{attribute 'no_assign'}
FUNCTION_BLOCK FB_IEDClient IMPLEMENTS I_ScsmAbortIndEventSink, I_ScsmAssociateCnfEventSink, I_ScsmGetServerDirectoryCnfEventSink, I_ScsmGetLogicalDeviceDirectoryCnfEventSink, I_ScsmGetLogicalNodeDirectoryCnfEventSink, I_ScsmGetDataValuesCnfEventSink, I_ScsmSetDataValuesCnfEventSink, I_ScsmReportIndEventSink, I_ScsmControlCnfEventSink, I_ScsmLastApplErrorIndEventSink, I_ScsmCommandTerminationIndEventSink
VAR_INPUT
	fbConnection		: FB_iec61850ClientClass := (ipAbortInd:=THIS^, ipAssociateCnf:=THIS^, ipGetServerDirectoryCnf:=THIS^, ipGetLogicalDeviceDirectoryCnf:=THIS^, ipGetLogicalNodeDirectoryCnf:=THIS^, ipGetDataValuesCnf:=THIS^, ipSetDataValuesCnf:=THIS^, ipReportInd:=THIS^, ipControlCnf:=THIS^, ipLastApplErrorInd:=THIS^, ipCommandTerminationInd:=THIS^);
END_VAR
VAR
	_bAbort				: BOOL; (* Rising edge activates AbortReq() command execution *)
	_bDisconnect		: BOOL; (* Rising edge activates ReleaseReq() command execution *)
	_bConnect			: BOOL; (* Rising edge activates AssociateReq() command execution *)
	_bReconnect			: BOOL := TRUE; (* TRUE => reconnect automatically *)
	_bReadAllData		: BOOL := TRUE; (* TRUE => read/refresh all data values on reconnect *)
	
	state				: BYTE;
	eState				: E_AsyncEnvironmentState; (* Environment state *)
	eLinkStatus			: E_ScsmLinkStatus; (* Network adapter link status *)
	bBusy				: BOOL; (* If TRUE => command execution is busy *)
	bSuccess			: BOOL;
	ipResult			: I_AsyncServiceResultClass;
	sLastErrorResult	: T_MaxString;
	fbAbortReason		: FB_ServiceErrorClass := (stError:=SUCCESS_EVENT);
	sLastAbortReason	: T_MaxString;
	nInvokeID			: UDINT;
	eServiceError		: E_AcsiServiceError; (* Latest OnXyzCnf() or OnXyzInd() event handler error *)
	nServiceError		: UDINT; (* Counts OnXyzCnf() and OnXyzInd() event handler errors *)
	nCmdError			: UDINT; (* Counts xyzReq() command errors *)
	sObjReference		: T_AcsiObjectReference; (* DATA object reference *)
	sCtrlReference		: T_AcsiObjectReference; (* CONTROLLABLE-DATA object reference *)
	
	bGetServerDirectory				: BOOL := TRUE; (* Rising edge enumerates logical-devices *)
	bGetLogicalDeviceDirectory		: BOOL := TRUE; (* Rising edge enumerates logical-nodes *)
	bGetLogicalNodeDirectory		: BOOL := TRUE; (* Rising edge enumerates "IEDMUnn/LLN0" data-sets *)
	bGetAllServerValues				: BOOL := TRUE; (* Rising edge reads all "IED" data attribute values *)
	bGetAllDataValues_LLN0_ST		: BOOL := TRUE; (* Rising edge reads all "IEDMUnn/LLN0.ST" data attribute values (having selected functional constraint) *)
	bGetDataValues_LLN0_ST_Beh		: BOOL := TRUE; (* Rising edge reads all "IEDMUnn/LLN0.ST.Beh" data attribute values (having selected functional constraint) *)
END_VAR

fbConnection.Execute();
eState:= fbConnection.eState;
eLinkStatus:= fbConnection.eLinkStatus;

CASE state OF
	0: (* Initial state *)
		IF _bAbort THEN (* Abort connection => execute AbortReq() command *)
			_bAbort:= FALSE;
			bSuccess:= fbConnection.AbortReq(ipReason:=fbAbortReason, ipSink:=0, ipResult=>ipResult);
			state:= SEL(bSuccess, 100, 1);
		ELSIF eState = E_AsyncEnvironmentState.Idle AND (_bConnect OR _bReconnect) THEN (* Open/establish connection => execute AssociateReq() command *)
			_bConnect:= FALSE;
			bGetAllServerValues:= SEL(_bReadAllData, bGetAllServerValues, TRUE);
			bSuccess:= fbConnection.AssociateReq(ipSink:=0, ipResult=>ipResult);
			state:= SEL(bSuccess, 100, 1);
		ELSIF eState = E_AsyncEnvironmentState.Established AND _bDisconnect THEN (* Close/release connection => execute ReleaseReq() command *)
			_bDisconnect:= FALSE;
			bSuccess:= fbConnection.ReleaseReq(ipSink:=0, ipResult=>ipResult);
			state:= SEL(bSuccess, 100, 1);
		ELSIF eState = E_AsyncEnvironmentState.Established THEN (* Connection established => exchange IED data *)
			state:= 10;
		END_IF
		_bConnect:= FALSE;
		_bDisconnect:= FALSE;
		(*==================================================================================================================================================================*)
	1: (* Wait for AbortReq() or ReleaseReq() or AssociateReq() command completion *)
		IF ipResult <> 0 THEN
			ipResult.Execute();
			IF NOT (bBusy:=ipResult.IsBusy()) THEN
				state:= SEL(ipResult.IsCompleted(), 100(* failed or aborted *), 0(* succeeded *));
			END_IF
		END_IF
		(*==================================================================================================================================================================*)
	10: (* Read/Write IED data *)
		IF bGetServerDirectory THEN (* Example => execute GetServerDirectoryReq() command *)
			bGetServerDirectory:= FALSE;
			bSuccess:= fbConnection.GetServerDirectoryReq(ipServer:=fbIED, eClass:=E_AcsiServerDirectoryClass.LogicalDevice, hUser:=0, ipSink:=0, nInvokeID=>nInvokeID, ipResult=>ipResult);
			state:= SEL(bSuccess, 100, 11);
		ELSIF bGetLogicalDeviceDirectory THEN (* Example => execute GetLogicalDeviceDirectoryReq() command *)
			bGetLogicalDeviceDirectory:= FALSE;
			bSuccess:= fbConnection.GetLogicalDeviceDirectoryReq(ipLogicalDevice:=fbIED.IEDMUnn, hUser:=0, ipSink:=0, nInvokeID=>nInvokeID, ipResult=>ipResult);
			state:= SEL(bSuccess, 100, 11);
		ELSIF bGetLogicalNodeDirectory THEN (* Example => execute GetLogicalNodeDirectoryReq() command *)
			bGetLogicalNodeDirectory:= FALSE;
			bSuccess:= fbConnection.GetLogicalNodeDirectoryReq(ipLogicalNode:=fbIED.IEDMUnn.LLN0, eClass:=E_AcsiLogicalNodeClass.DataSet, hUser:=0, ipSink:=0, nInvokeID=>nInvokeID, ipResult=>ipResult);
			state:= SEL(bSuccess, 100, 11);
		ELSIF bGetAllServerValues THEN (* Example => execute GetAllServerValues() command *)
			bGetAllServerValues:= FALSE;
			bSuccess:= fbConnection.GetAllServerValuesReq(ipServer:=fbIED, hUser:=0, ipSink:=0, nInvokeID=>nInvokeID, ipResult=>ipResult);
			state:= SEL(bSuccess, 100, 11);
		ELSIF bGetAllDataValues_LLN0_ST THEN (* Example => execute GetAllDataValuesReq() command *)
			bGetAllDataValues_LLN0_ST:= FALSE;
			bSuccess:= fbConnection.GetAllDataValuesReq(ipLogicalNode:=fbIED.IEDMUnn.LLN0, eFc:=E_AcsiFc.ST_, hUser:=0, ipSink:=0, nInvokeID=>nInvokeID, ipResult=>ipResult);
			state:= SEL(bSuccess, 100, 11);
		ELSIF bGetDataValues_LLN0_ST_Beh THEN (* Example => execute GetDataValuesReq() command *)
			bGetDataValues_LLN0_ST_Beh:= FALSE;
			bSuccess:= fbConnection.GetDataValuesReq(ipData:=fbIED.IEDMUnn.LLN0.Beh, eFc:=E_AcsiFc.ST_, hUser:=0, ipSink:=0, nInvokeID=>nInvokeID, ipResult=>ipResult);
			state:= SEL(bSuccess, 100, 11);
		ELSE
			state:= 0;
		END_IF
		(*==================================================================================================================================================================*)
	11: (* Wait for GetServerDirectoryReq(), GetLogicalDeviceDirectoryReq(), GetLogicalNodeDirectoryReq(), GetAllServerValuesReq(), GetAllDataValuesReq() or GetDataValuesReq() command completion *)
		IF ipResult <> 0 THEN
			ipResult.Execute();
			IF NOT (bBusy:=ipResult.IsBusy()) THEN
				state:= SEL(ipResult.IsCompleted(), 100(* failed or aborted *), 0(* succeeded *));
			END_IF
		END_IF
		(*==================================================================================================================================================================*)
	100: (* Error state *)
		state:= 0;
		IF ipResult <> 0 THEN
			nCmdError:= nCmdError + 1;
			sLastErrorResult:= ipResult.Dump();
		END_IF
END_CASE

PROPERTY bAbort : BOOL
SET
_bAbort:= bAbort;
END_SET
END_PROPERTY

PROPERTY bConnect : BOOL
SET
_bConnect:= bConnect;
END_SET
END_PROPERTY

PROPERTY bDisconnect : BOOL
SET
_bDisconnect:= bDisconnect;
END_SET
END_PROPERTY

PROPERTY bReconnect : BOOL
SET
_bReconnect:= bReconnect;
END_SET
END_PROPERTY

{attribute 'analysis' := '-33'}
(* This method receives IEC61850::Abort.ind primitive. *)
METHOD OnAbortInd
VAR_INPUT
	ipAA		: I_ScsmAssociationClass; (* Application association. If = 0 => optional. *)
	bPAbort		: BOOL; (* TRUE => P-Abort.request(), issued by provider, FALSE => Abort.request(), issued by user. *)
	ipReason	: I_ServiceErrorClass; (* Abort reason. *)
	ipData		: I_BaseStreamClass; (* Optional data. If = 0 => default, no data. *)
END_VAR
VAR
END_VAR
IF ipReason <> 0 THEN
	sLastAbortReason:= ipReason.Dump();
END_IF
END_METHOD

{attribute 'analysis' := '-33'}
(* This method receives IEC61850::Associate.cnf primitive. *)
METHOD OnAssociateCnf
VAR_INPUT
	ipAA			: I_ScsmAssociationClass; (* Application association. If = 0 => optional. *)
	eError			: E_AcsiServiceError; (* Error code *)
END_VAR
VAR
END_VAR
sLastAbortReason:= '';
sLastErrorResult:= '';
END_METHOD

{attribute 'analysis' := '-33'}
(* This method receives buffered IEC61850::Report.ind primitive. *)
METHOD OnBufferedReportInd
VAR_INPUT
	ipAA		: I_ScsmAssociationClass; (* Application association. If = 0 => optional. *)
	info		: ST_ScsmReportEventInfo;
	ipBrcb		: I_AcsiCommonBufferedReportControlBlockClass; (* Interface pointer to BRCB object. *)
	ipDataSet	: I_AcsiCommonDataSetClass; (* Interface pointer to data-set object. *)
	ipData		: I_AcsiCommonDataClass; (* Interface pointer to reported data object. *)
	eFc			: E_AcsiFc; (* Functional constraint of reported data. *)
	eError		: E_AcsiServiceError; (* Data access error code. *)
END_VAR
VAR
END_VAR
IF eError <> E_AcsiServiceError.NoError THEN
	eServiceError:= eError;
	nServiceError:= nServiceError + 1;
END_IF
IF ipData <> 0 THEN
	sObjReference:= ipData.GetObjectReference();
END_IF
END_METHOD

{attribute 'analysis' := '-33'}
(* This method receives IEC61850::CommandTermination.ind primitive. *)
METHOD OnCommandTerminationInd
VAR_INPUT
	ipAA		: I_ScsmAssociationClass; (* Application association. If = 0 => optional. *)
	info		: ST_ScsmCommandTerminationEventInfo;
	ipCtrl		: I_AcsiCommonControllableDataClass; (* Interface pointer to controllable data object. *)
	ipData		: I_AcsiCommonDataClass; (* Interface pointer to Oper/Cancel/SBO or SBOw data object. *)
	eFc			: E_AcsiFc; (* Functional constraint (CO). *)
	eError		: E_AcsiServiceError; (* Error code. *)
END_VAR
VAR
END_VAR
IF eError <> E_AcsiServiceError.NoError THEN
	eServiceError:= eError;
	nServiceError:= nServiceError + 1;
END_IF
IF ipCtrl <> 0 THEN
	sCtrlReference:= ipCtrl.GetObjectReference();
END_IF
IF ipData <> 0 THEN
	sObjReference:= ipData.GetObjectReference();
END_IF
END_METHOD

{attribute 'analysis' := '-33'}
(* This method receives IEC61850::Control[Select|Operate|SelectWithValue|Cancel].cnf primitive. *)
METHOD OnControlCnf
VAR_INPUT
	ipAA		: I_ScsmAssociationClass; (* Application association. If = 0 => optional. *)
	info		: ST_ScsmConfirmedEventInfo;
	ipCtrl		: I_AcsiCommonControllableDataClass; (* Interface pointer to controllable data object. *)
	ipData		: I_AcsiCommonDataClass; (* Interface pointer to Oper/Cancel/SBO or SBOw data object. *)
	eFc			: E_AcsiFc; (* Functional constraint (CO). *)
	eError		: E_AcsiServiceError; (* Write/Read data access error code. *)
END_VAR
VAR
END_VAR
IF eError <> E_AcsiServiceError.NoError THEN
	eServiceError:= eError;
	nServiceError:= nServiceError + 1;
END_IF
IF ipCtrl <> 0 THEN
	sCtrlReference:= ipCtrl.GetObjectReference();
END_IF
IF ipData <> 0 THEN
	sObjReference:= ipData.GetObjectReference();
END_IF
END_METHOD

{attribute 'analysis' := '-33'}
(* This method receives IEC61850::GetDataValues.cnf primitive. *)
METHOD OnGetDataValuesCnf
VAR_INPUT
	ipAA		: I_ScsmAssociationClass; (* Application association. If = 0 => optional. *)
	info		: ST_ScsmConfirmedEventInfo;
	ipData		: I_AcsiCommonDataClass; (* Interface pointer to read data object. *)
	eFc			: E_AcsiFc; (* Functional constraint of read data. *)
	eError		: E_AcsiServiceError; (* Data access error code. *)
END_VAR
VAR
END_VAR
IF eError <> E_AcsiServiceError.NoError THEN
	eServiceError:= eError;
	nServiceError:= nServiceError + 1;
END_IF
IF ipData <> 0 THEN
	sObjReference:= ipData.GetObjectReference();
END_IF
END_METHOD

{attribute 'analysis' := '-33'}
(* This method receives IEC61850::GetLogicalDeviceDirectory.cnf primitive. *)
METHOD OnGetLogicalDeviceDirectoryCnf
VAR_INPUT
	ipAA				: I_ScsmAssociationClass; (* Application association. If = 0 => optional. *)
	info				: ST_ScsmConfirmedEventInfo;
	ipLogicalDevice		: I_AcsiCommonLogicalDeviceClass; (* Interface pointer to logical-device object. *)
	sObjectReference	: T_AcsiObjectReference;
	eError				: E_AcsiServiceError; (* Logical-device class access error code. *)
END_VAR
VAR
END_VAR
IF eError <> E_AcsiServiceError.NoError THEN
	eServiceError:= eError;
	nServiceError:= nServiceError + 1;
END_IF
sObjReference:= sObjectReference;
END_METHOD

{attribute 'analysis' := '-33'}
(* This method receives IEC61850::GetLogicalNodeDirectory.cnf primitive. *)
METHOD OnGetLogicalNodeDirectoryCnf
VAR_INPUT
	ipAA				: I_ScsmAssociationClass; (* Application association. If = 0 => optional. *)
	info				: ST_ScsmConfirmedEventInfo;
	ipLogicalNode		: I_AcsiCommonLogicalNodeClass; (* Interface pointer to logical-node object. *)
	eClass				: E_AcsiLogicalNodeClass; (* Logical-node directory class (BRCB, URCB, DATA-SET, ... ). *)
	sObjectReference	: T_AcsiObjectReference;
	eError				: E_AcsiServiceError; (* Logical-node class access error code. *)
END_VAR
VAR
END_VAR
IF eError <> E_AcsiServiceError.NoError THEN
	eServiceError:= eError;
	nServiceError:= nServiceError + 1;
END_IF
sObjReference:= sObjectReference;
END_METHOD

{attribute 'analysis' := '-33'}
(* This method receives IEC61850::GetServerDirectory.cnf primitive. *)
METHOD OnGetServerDirectoryCnf
VAR_INPUT
	ipAA				: I_ScsmAssociationClass; (* Application association. If = 0 => optional. *)
	info				: ST_ScsmConfirmedEventInfo;
	ipServer			: I_AcsiCommonIntelligentElectronicDeviceClass; (* Interface pointer to server object. *)
	eClass				: E_AcsiServerDirectoryClass; (* Server directory class (logical-device or file). *)
	sObjectReference	: T_AcsiObjectReference;
	eError				: E_AcsiServiceError; (* Server class (logical-device) access error code. *)
END_VAR
VAR
END_VAR
IF eError <> E_AcsiServiceError.NoError THEN
	eServiceError:= eError;
	nServiceError:= nServiceError + 1;
END_IF
sObjReference:= sObjectReference;
END_METHOD

{attribute 'analysis' := '-33'}
(* This method receives IEC61850::LastApplError.ind primitive. *)
METHOD OnLastApplErrorInd
VAR_INPUT
	ipAA		: I_ScsmAssociationClass; (* Application association. If = 0 => optional. *)
	info		: ST_ScsmAdditionalCauseDiagnosticEventInfo;
	ipCtrl		: I_AcsiCommonControllableDataClass; (* Interface pointer to controllable data object. *)
	eError		: E_AcsiServiceError; (* Error code. *)
END_VAR
VAR
END_VAR
IF eError <> E_AcsiServiceError.NoError THEN
	eServiceError:= eError;
	nServiceError:= nServiceError + 1;
END_IF
IF ipCtrl <> 0 THEN
	sCtrlReference:= ipCtrl.GetObjectReference();
END_IF
END_METHOD

{attribute 'analysis' := '-33'}
(* This method receives IEC61850::SetDataValues.cnf primitive. *)
METHOD OnSetDataValuesCnf
VAR_INPUT
	ipAA		: I_ScsmAssociationClass; (* Application association. If = 0 => optional. *)
	info		: ST_ScsmConfirmedEventInfo;
	ipData		: I_AcsiCommonDataClass; (* Interface pointer to written data object. *)
	eFc			: E_AcsiFc; (* Functional constraint of written data. *)
	eError		: E_AcsiServiceError; (* Data access error code. *)
END_VAR
VAR
END_VAR
IF eError <> E_AcsiServiceError.NoError THEN
	eServiceError:= eError;
	nServiceError:= nServiceError + 1;
END_IF
IF ipData <> 0 THEN
	sObjReference:= ipData.GetObjectReference();
END_IF
END_METHOD

{attribute 'analysis' := '-33'}
(* This method receives unbuffered IEC61850::Report.ind primitive. *)
METHOD OnUnbufferedReportInd
VAR_INPUT
	ipAA		: I_ScsmAssociationClass; (* Application association. If = 0 => optional. *)
	info		: ST_ScsmReportEventInfo;
	ipUrcb		: I_AcsiCommonUnbufferedReportControlBlockClass; (* Interface pointer to URCB object. *)
	ipDataSet	: I_AcsiCommonDataSetClass; (* Interface pointer to dataset object. *)
	ipData		: I_AcsiCommonDataClass; (* Interface pointer to reported data object. *)
	eFc			: E_AcsiFc; (* Functional constraint of reported data. *)
	eError		: E_AcsiServiceError; (* Data access error code. *)
END_VAR
VAR
END_VAR
IF eError <> E_AcsiServiceError.NoError THEN
	eServiceError:= eError;
	nServiceError:= nServiceError + 1;
END_IF
IF ipData <> 0 THEN
	sObjReference:= ipData.GetObjectReference();
END_IF
END_METHOD

END_FUNCTION_BLOCK
